| IBIS file useshx1xxac.ibs created by s2ibis3 verion 1.1
| North Carolina State University, ERL, 2006
| This Model is valid for Commercial Temperature Range 0C<=Tc<=95C
| Valid for DDR3-800/1066/1333/1600/1866 operation
| Part Number   VDD/VDDQ   Package   Architecture
| SCE15H1G160AF   1.5 +0.1/-0.1 96-Ball FBGA   64Meg x 16
| SCE15H1G800AF   1.5 +0.1/-0.1 78-Ball FBGA   128Meg x 8
| SCX15H512160AF   1.5 +0.1/-0.1 96-Ball FBGA   32Meg x 16
| SCX15H512800AF   1.5 +0.1/-0.1 78-Ball FBGA   64Meg x 8
[IBIS Ver]   3.2
[File name]  useshx1xxac.ibs
[File Rev]   1.2
[Date]   2016-10-26
[Source]   Simulation of a silicon level SPICE model
[Notes]   IBIS Characteristics for I/O Buffer
   IBIS Model Revision History:
Rev 1.1: 2014-07-22
   - IBIS model file initial creation
Rev 1.2: 2016-10-26
   - Updata company and other informations
   - Updata Rising/Falling Waveform for High speed
   - Updata power clamp of ODT_120/ODT_60/ODT_40/ODT_30/ODT_20
   - Updata package RLC value
[disclaimer] The IBIS models are for modeling purpose only and are
   subject to change without any notice. UniIC is not
   responsible for any problems the models may cause.
[Copyright]  Copyright 2009 UniIC Semiconductors Corp. All rights reserved
|   Component SCE15H1G160AF
[Component]   SCE15H1G160AF
[Manufacturer]  UniIC Semiconductors Corp.
| All balls excluding NC, POWER and GND (R[Ohm], L[H], C[F])
[Package]   | 96-Ball FBGA
|Variable   typ   min   max
R_pkg   4.62E-01   3.18E-01   5.65E-01
L_pkg   1.73E-09   1.10E-09   2.38E-09
C_pkg   5.30E-13   3.68E-13   7.38E-13
[Pin]   signal_name   model_name   R_pin   L_pin   C_pin
A1   VDDQ   POWER   NA   NA   NA
A2   DQU5   DQ   5.56E-01   1.93E-09   6.92E-13
A3   DQU7   DQ   4.86E-01   1.59E-09   6.10E-13
A7   DQU4   DQ   4.57E-01   1.38E-09   6.09E-13
A8   VDDQ   POWER   NA   NA   NA
A9   VSS   GND   NA   NA   NA
B1   VSSQ   GND   NA   NA   NA
B2   VDD   POWER   NA   NA   NA
B3   VSS   GND   NA   NA   NA
B7   DQSU#   DQ   5.07E-01   1.70E-09   5.10E-13
B8   DQU6   DQ   5.35E-01   1.74E-09   7.38E-13
B9   VSSQ   GND   NA   NA   NA
C1   VDDQ   POWER   NA   NA   NA
C2   DQU3   DQ   5.65E-01   1.76E-09   7.07E-13
C3   DQU1   DQ   4.98E-01   1.59E-09   6.47E-13
C7   DQSU   DQ   5.17E-01   1.87E-09   5.43E-13
C8   DQU2   DQ   4.97E-01   1.58E-09   5.57E-13
C9   VDDQ   POWER   NA   NA   NA
D1   VSSQ   GND   NA   NA   NA
D2   VDDQ   POWER   NA   NA   NA
D3   DMU   DM   4.84E-01   1.56E-09   6.30E-13
D7   DQU0   DQ   4.67E-01   1.57E-09   5.05E-13
D8   VSSQ   GND   NA   NA   NA
D9   VDD   POWER   NA   NA   NA
E1   VSS   GND   NA   NA   NA
E2   VSSQ   GND   NA   NA   NA
E3   DQL0   DQ   4.79E-01   1.40E-09   4.50E-13
E7   DML   DM   4.78E-01   1.54E-09   6.77E-13
E8   VSSQ   GND   NA   NA   NA
E9   VDDQ   POWER   NA   NA   NA
F1   VDDQ   POWER   NA   NA   NA
F2   DQL2   DQ   4.68E-01   1.62E-09   6.68E-13
F3   DQSL   DQ   4.57E-01   1.58E-09   4.57E-13
F7   DQL1   DQ   4.61E-01   1.63E-09   5.21E-13
F8   DQL3   DQ   5.04E-01   1.79E-09   6.87E-13
F9   VSSQ   GND   NA   NA   NA
G1   VSSQ   GND   NA   NA   NA
G2   DQL6   DQ   4.89E-01   1.50E-09   6.81E-13
G3   DQSL#   DQ   4.62E-01   1.55E-09   4.40E-13
G7   VDD   POWER   NA   NA   NA
G8   VSS   GND   NA   NA   NA
G9   VSSQ   GND   NA   NA   NA
H1   VREFDQ   POWER   NA   NA   NA
H2   VDDQ   POWER   NA   NA   NA
H3   DQL4   DQ   4.85E-01   1.58E-09   4.54E-13
H7   DQL7   DQ   4.57E-01   1.57E-09   4.72E-13
H8   DQL5   DQ   5.42E-01   1.77E-09   6.76E-13
H9   VDDQ   POWER   NA   NA   NA
J2   VSS   GND   NA   NA   NA
J3   RAS#   CLKCA_RCV   4.11E-01   1.55E-09   3.80E-13
J7   CK   CLKCA_RCV   4.24E-01   1.47E-09   3.68E-13
J8   VSS   GND   NA   NA   NA
K1   ODT   CLKCA_RCV   4.58E-01   1.94E-09   5.18E-13
K2   VDD   POWER   NA   NA   NA
K3   CAS#   CLKCA_RCV   3.18E-01   1.10E-09   4.11E-13
K7   CK#   CLKCA_RCV   4.31E-01   1.48E-09   3.87E-13
K8   VDD   POWER   NA   NA   NA
K9   CKE   CLKCA_RCV   4.57E-01   1.89E-09   4.77E-13
L2   CS#   CLKCA_RCV   4.36E-01   1.93E-09   5.07E-13
L3   WE#   CLKCA_RCV   4.32E-01   1.83E-09   4.90E-13
L7   A10   CLKCA_RCV   3.83E-01   1.62E-09   3.69E-13
L8   ZQ   NC   NA   NA   NA
M1   VSS   GND   NA   NA   NA
M2   BA0   CLKCA_RCV   4.00E-01   1.64E-09   4.95E-13
M3   BA2   CLKCA_RCV   4.44E-01   1.78E-09   4.47E-13
M8   VREFCA   POWER   NA   NA   NA
M9   VSS   GND   NA   NA   NA
N1   VDD   POWER   NA   NA   NA
N2   A3   CLKCA_RCV   4.56E-01   2.02E-09   4.33E-13
N3   A0   CLKCA_RCV   4.36E-01   1.84E-09   5.69E-13
N7   A12   CLKCA_RCV   3.99E-01   1.63E-09   5.01E-13
N8   BA1   CLKCA_RCV   4.64E-01   2.16E-09   4.55E-13
N9   VDD   POWER   NA   NA   NA
P1   VSS   GND   NA   NA   NA
P2   A5   CLKCA_RCV   4.19E-01   2.02E-09   5.57E-13
P3   A2   CLKCA_RCV   4.74E-01   1.94E-09   4.53E-13
P7   A1   CLKCA_RCV   4.35E-01   1.87E-09   4.43E-13
P8   A4   CLKCA_RCV   4.15E-01   1.88E-09   5.10E-13
P9   VSS   GND   NA   NA   NA
R1   VDD   POWER   NA   NA   NA
R2   A7   CLKCA_RCV   4.68E-01   1.94E-09   4.71E-13
R3   A9   CLKCA_RCV   4.27E-01   1.66E-09   5.18E-13
R7   A11   CLKCA_RCV   4.71E-01   1.94E-09   5.10E-13
R8   A6   CLKCA_RCV   4.71E-01   1.83E-09   4.71E-13
R9   VDD   POWER   NA   NA   NA
T1   VSS   GND   NA   NA   NA
T2   RESET#   CLKCA_RCV   4.79E-01   2.35E-09   7.31E-13
T3   A13   CLKCA_RCV   4.30E-01   1.76E-09   4.55E-13
T7   A14   CLKCA_RCV   4.33E-01   1.73E-09   5.40E-13
T8   A8   CLKCA_RCV   5.20E-01   2.38E-09   5.59E-13
T9   VSS   GND   NA   NA   NA
|*****************************  Diff Pin  *************************************
[Diff Pin]  inv_pin  vdiff   tdelay_typ  tdelay_min  tdelay_max
C7   B7   0.25000V   NA   NA   NA
F3   G3   0.25000V   NA   NA   NA
J7   K7   0.25000V   NA   NA   NA
|   Component SCE15H1G800AF
[Component]   SCE15H1G800AF
[Manufacturer]  UniIC Semiconductors Corp.
[Package]   | 78-Ball FBGA
|Variable   typ   min   max
R_pkg   3.88E-01   2.67E-01   5.49E-01
L_pkg   1.55E-09   1.21E-09   2.00E-09
C_pkg   5.15E-13   2.92E-13   7.34E-13
[Pin]   signal_name   model_name   R_pin   L_pin   C_pin
A1   VSS   GND   NA   NA   NA
A2   VDD   POWER   NA   NA   NA
A7   NU_TDQS#   NU_TDQS#   5.42E-01   1.89E-09   6.76E-13
A8   VSS   GND   NA   NA   NA
A9   VDD   POWER   NA   NA   NA
B1   VSS   GND   NA   NA   NA
B2   VSSQ   GND   NA   NA   NA
B3   DQ0   DQ   4.03E-01   1.53E-09   5.94E-13
B7   DM_TDQS   DM_TDQS   4.61E-01   1.83E-09   6.42E-13
B8   VSSQ   GND   NA   NA   NA
B9   VDDQ   POWER   NA   NA   NA
C1   VDDQ   POWER   NA   NA   NA
C2   DQ2   DQ   5.07E-01   1.89E-09   7.34E-13
C3   DQS   DQ   3.96E-01   1.55E-09   5.43E-13
C7   DQ1   DQ   4.34E-01   1.72E-09   5.27E-13
C8   DQ3   DQ   4.21E-01   1.77E-09   6.68E-13
C9   VSSQ   GND   NA   NA   NA
D1   VSSQ   GND   NA   NA   NA
D2   DQ6   DQ   5.49E-01   1.81E-09   6.19E-13
D3   DQS#   DQ   4.15E-01   1.63E-09   5.34E-13
D7   VDD   POWER   NA   NA   NA
D8   VSS   GND   NA   NA   NA
D9   VSSQ   GND   NA   NA   NA
E1   VREFDQ   POWER   NA   NA   NA
E2   VDDQ   POWER   NA   NA   NA
E3   DQ4   DQ   4.95E-01   1.56E-09   5.48E-13
E7   DQ7   DQ   4.13E-01   1.44E-09   4.60E-13
E8   DQ5   DQ   5.04E-01   1.56E-09   5.90E-13
E9   VDDQ   POWER   NA   NA   NA
F2   VSS   GND   NA   NA   NA
F3   RAS#   CLKCA_RCV   3.73E-01   1.42E-09   5.66E-13
F7   CK   CLKCA_RCV   3.22E-01   1.30E-09   4.89E-13
F8   VSS   GND   NA   NA   NA
G1   ODT   CLKCA_RCV   4.68E-01   2.00E-09   6.71E-13
G2   VDD   POWER   NA   NA   NA
G3   CAS#   CLKCA_RCV   3.75E-01   1.60E-09   4.41E-13
G7   CK#   CLKCA_RCV   3.24E-01   1.21E-09   4.51E-13
G8   VDD   POWER   NA   NA   NA
G9   CKE   CLKCA_RCV   4.14E-01   1.86E-09   7.10E-13
H2   CS#   CLKCA_RCV   3.75E-01   1.70E-09   5.45E-13
H3   WE#   CLKCA_RCV   3.53E-01   1.56E-09   3.77E-13
H7   A10   CLKCA_RCV   3.46E-01   1.38E-09   3.01E-13
H8   ZQ   NC   NA   NA   NA
J1   VSS   GND   NA   NA   NA
J2   BA0   CLKCA_RCV   3.35E-01   1.43E-09   5.84E-13
J3   BA2   CLKCA_RCV   3.55E-01   1.44E-09   5.18E-13
J8   VREFCA   POWER   NA   NA   NA
J9   VSS   GND   NA   NA   NA
K1   VDD   POWER   NA   NA   NA
K2   A3   CLKCA_RCV   3.89E-01   1.55E-09   4.28E-13
K3   A0   CLKCA_RCV   3.42E-01   1.52E-09   2.92E-13
K7   A12   CLKCA_RCV   3.25E-01   1.26E-09   4.48E-13
K8   BA1   CLKCA_RCV   3.14E-01   1.33E-09   4.58E-13
K9   VDD   POWER   NA   NA   NA
L1   VSS   GND   NA   NA   NA
L2   A5   CLKCA_RCV   3.29E-01   1.36E-09   4.52E-13
L3   A2   CLKCA_RCV   3.47E-01   1.59E-09   3.74E-13
L7   A1   CLKCA_RCV   3.45E-01   1.55E-09   4.31E-13
L8   A4   CLKCA_RCV   3.87E-01   1.46E-09   5.27E-13
L9   VSS   GND   NA   NA   NA
M1   VDD   POWER   NA   NA   NA
M2   A7   CLKCA_RCV   3.58E-01   1.50E-09   4.81E-13
M3   A9   CLKCA_RCV   3.32E-01   1.31E-09   3.74E-13
M7   A11   CLKCA_RCV   3.67E-01   1.54E-09   4.33E-13
M8   A6   CLKCA_RCV   3.71E-01   1.43E-09   5.17E-13
M9   VDD   POWER   NA   NA   NA
N1   VSS   GND   NA   NA   NA
N2   RESET#   CLKCA_RCV   2.67E-01   1.54E-09   6.32E-13
N3   A13   CLKCA_RCV   3.36E-01   1.31E-09   4.39E-13
N8   A8   CLKCA_RCV   3.43E-01   1.50E-09   5.05E-13
N9   VSS   GND   NA   NA   NA
|*****************************  Diff Pin  *************************************
[Diff Pin]  inv_pin  vdiff   tdelay_typ  tdelay_min  tdelay_max
F7   G7   0.25000V   NA   NA   NA
C3   D3   0.25000V   NA   NA   NA
|B7   A7   0.25000V   NA   NA   NA
|pin B7 and A7 are differential I/O only When TDQS/TDQS#
|is enabled via Mode Register A11=1 in MR1
|If TDQS is disabled, then B7 (DM) is a single
|ended INPUT with ODT and A7 is a NC
|   Component SCX15H512160AF
[Component]   SCX15H512160AF
[Manufacturer]  UniIC Semiconductors Corp.
| All balls excluding NC, POWER and GND (R[Ohm], L[H], C[F])
[Package]   | 96-Ball FBGA
|Variable   typ   min   max
R_pkg   4.62E-01   3.18E-01   5.65E-01
L_pkg   1.73E-09   1.10E-09   2.38E-09
C_pkg   5.30E-13   3.68E-13   7.38E-13
[Pin]   signal_name   model_name   R_pin   L_pin   C_pin
A1   VDDQ   POWER   NA   NA   NA
A2   DQU5   DQ   5.56E-01   1.93E-09   6.92E-13
A3   DQU7   DQ   4.86E-01   1.59E-09   6.10E-13
A7   DQU4   DQ   4.57E-01   1.38E-09   6.09E-13
A8   VDDQ   POWER   NA   NA   NA
A9   VSS   GND   NA   NA   NA
B1   VSSQ   GND   NA   NA   NA
B2   VDD   POWER   NA   NA   NA
B3   VSS   GND   NA   NA   NA
B7   DQSU#   DQ   5.07E-01   1.70E-09   5.10E-13
B8   DQU6   DQ   5.35E-01   1.74E-09   7.38E-13
B9   VSSQ   GND   NA   NA   NA
C1   VDDQ   POWER   NA   NA   NA
C2   DQU3   DQ   5.65E-01   1.76E-09   7.07E-13
C3   DQU1   DQ   4.98E-01   1.59E-09   6.47E-13
C7   DQSU   DQ   5.17E-01   1.87E-09   5.43E-13
C8   DQU2   DQ   4.97E-01   1.58E-09   5.57E-13
C9   VDDQ   POWER   NA   NA   NA
D1   VSSQ   GND   NA   NA   NA
D2   VDDQ   POWER   NA   NA   NA
D3   DMU   DM   4.84E-01   1.56E-09   6.30E-13
D7   DQU0   DQ   4.67E-01   1.57E-09   5.05E-13
D8   VSSQ   GND   NA   NA   NA
D9   VDD   POWER   NA   NA   NA
E1   VSS   GND   NA   NA   NA
E2   VSSQ   GND   NA   NA   NA
E3   DQL0   DQ   4.79E-01   1.40E-09   4.50E-13
E7   DML   DM   4.78E-01   1.54E-09   6.77E-13
E8   VSSQ   GND   NA   NA   NA
E9   VDDQ   POWER   NA   NA   NA
F1   VDDQ   POWER   NA   NA   NA
F2   DQL2   DQ   4.68E-01   1.62E-09   6.68E-13
F3   DQSL   DQ   4.57E-01   1.58E-09   4.57E-13
F7   DQL1   DQ   4.61E-01   1.63E-09   5.21E-13
F8   DQL3   DQ   5.04E-01   1.79E-09   6.87E-13
F9   VSSQ   GND   NA   NA   NA
G1   VSSQ   GND   NA   NA   NA
G2   DQL6   DQ   4.89E-01   1.50E-09   6.81E-13
G3   DQSL#   DQ   4.62E-01   1.55E-09   4.40E-13
G7   VDD   POWER   NA   NA   NA
G8   VSS   GND   NA   NA   NA
G9   VSSQ   GND   NA   NA   NA
H1   VREFDQ   POWER   NA   NA   NA
H2   VDDQ   POWER   NA   NA   NA
H3   DQL4   DQ   4.85E-01   1.58E-09   4.54E-13
H7   DQL7   DQ   4.57E-01   1.57E-09   4.72E-13
H8   DQL5   DQ   5.42E-01   1.77E-09   6.76E-13
H9   VDDQ   POWER   NA   NA   NA
J2   VSS   GND   NA   NA   NA
J3   RAS#   CLKCA_RCV   4.11E-01   1.55E-09   3.80E-13
J7   CK   CLKCA_RCV   4.24E-01   1.47E-09   3.68E-13
J8   VSS   GND   NA   NA   NA
K1   ODT   CLKCA_RCV   4.58E-01   1.94E-09   5.18E-13
K2   VDD   POWER   NA   NA   NA
K3   CAS#   CLKCA_RCV   3.18E-01   1.10E-09   4.11E-13
K7   CK#   CLKCA_RCV   4.31E-01   1.48E-09   3.87E-13
K8   VDD   POWER   NA   NA   NA
K9   CKE   CLKCA_RCV   4.57E-01   1.89E-09   4.77E-13
L2   CS#   CLKCA_RCV   4.36E-01   1.93E-09   5.07E-13
L3   WE#   CLKCA_RCV   4.32E-01   1.83E-09   4.90E-13
L7   A10   CLKCA_RCV   3.83E-01   1.62E-09   3.69E-13
L8   ZQ   NC   NA   NA   NA
M1   VSS   GND   NA   NA   NA
M2   BA0   CLKCA_RCV   4.00E-01   1.64E-09   4.95E-13
M3   BA2   CLKCA_RCV   4.44E-01   1.78E-09   4.47E-13
M8   VREFCA   POWER   NA   NA   NA
M9   VSS   GND   NA   NA   NA
N1   VDD   POWER   NA   NA   NA
N2   A3   CLKCA_RCV   4.56E-01   2.02E-09   4.33E-13
N3   A0   CLKCA_RCV   4.36E-01   1.84E-09   5.69E-13
N7   A12   CLKCA_RCV   3.99E-01   1.63E-09   5.01E-13
N8   BA1   CLKCA_RCV   4.64E-01   2.16E-09   4.55E-13
N9   VDD   POWER   NA   NA   NA
P1   VSS   GND   NA   NA   NA
P2   A5   CLKCA_RCV   4.19E-01   2.02E-09   5.57E-13
P3   A2   CLKCA_RCV   4.74E-01   1.94E-09   4.53E-13
P7   A1   CLKCA_RCV   4.35E-01   1.87E-09   4.43E-13
P8   A4   CLKCA_RCV   4.15E-01   1.88E-09   5.10E-13
P9   VSS   GND   NA   NA   NA
R1   VDD   POWER   NA   NA   NA
R2   A7   CLKCA_RCV   4.68E-01   1.94E-09   4.71E-13
R3   A9   CLKCA_RCV   4.27E-01   1.66E-09   5.18E-13
R7   A11   CLKCA_RCV   4.71E-01   1.94E-09   5.10E-13
R8   A6   CLKCA_RCV   4.71E-01   1.83E-09   4.71E-13
R9   VDD   POWER   NA   NA   NA
T1   VSS   GND   NA   NA   NA
T2   RESET#   CLKCA_RCV   4.79E-01   2.35E-09   7.31E-13
T3   A13   CLKCA_RCV   4.30E-01   1.76E-09   4.55E-13
T7   A14   CLKCA_RCV   4.33E-01   1.73E-09   5.40E-13
T8   A8   CLKCA_RCV   5.20E-01   2.38E-09   5.59E-13
T9   VSS   GND   NA   NA   NA
|*****************************  Diff Pin  *************************************
[Diff Pin]  inv_pin  vdiff   tdelay_typ  tdelay_min  tdelay_max
C7   B7   0.25000V   NA   NA   NA
F3   G3   0.25000V   NA   NA   NA
J7   K7   0.25000V   NA   NA   NA
|   Component SCX15H512800AF
[Component]   SCX15H512800AF
[Manufacturer]  UniIC Semiconductors Corp.
[Package]   | 78-Ball FBGA
|Variable   typ   min   max
R_pkg   3.88E-01   2.67E-01   5.49E-01
L_pkg   1.55E-09   1.21E-09   2.00E-09
C_pkg   5.15E-13   2.92E-13   7.34E-13
[Pin]   signal_name   model_name   R_pin   L_pin   C_pin
A1   VSS   GND   NA   NA   NA
A2   VDD   POWER   NA   NA   NA
A7   NU_TDQS#   NU_TDQS#   5.42E-01   1.89E-09   6.76E-13
A8   VSS   GND   NA   NA   NA
A9   VDD   POWER   NA   NA   NA
B1   VSS   GND   NA   NA   NA
B2   VSSQ   GND   NA   NA   NA
B3   DQ0   DQ   4.03E-01   1.53E-09   5.94E-13
B7   DM_TDQS   DM_TDQS   4.61E-01   1.83E-09   6.42E-13
B8   VSSQ   GND   NA   NA   NA
B9   VDDQ   POWER   NA   NA   NA
C1   VDDQ   POWER   NA   NA   NA
C2   DQ2   DQ   5.07E-01   1.89E-09   7.34E-13
C3   DQS   DQ   3.96E-01   1.55E-09   5.43E-13
C7   DQ1   DQ   4.34E-01   1.72E-09   5.27E-13
C8   DQ3   DQ   4.21E-01   1.77E-09   6.68E-13
C9   VSSQ   GND   NA   NA   NA
D1   VSSQ   GND   NA   NA   NA
D2   DQ6   DQ   5.49E-01   1.81E-09   6.19E-13
D3   DQS#   DQ   4.15E-01   1.63E-09   5.34E-13
D7   VDD   POWER   NA   NA   NA
D8   VSS   GND   NA   NA   NA
D9   VSSQ   GND   NA   NA   NA
E1   VREFDQ   POWER   NA   NA   NA
E2   VDDQ   POWER   NA   NA   NA
E3   DQ4   DQ   4.95E-01   1.56E-09   5.48E-13
E7   DQ7   DQ   4.13E-01   1.44E-09   4.60E-13
E8   DQ5   DQ   5.04E-01   1.56E-09   5.90E-13
E9   VDDQ   POWER   NA   NA   NA
F2   VSS   GND   NA   NA   NA
F3   RAS#   CLKCA_RCV   3.73E-01   1.42E-09   5.66E-13
F7   CK   CLKCA_RCV   3.22E-01   1.30E-09   4.89E-13
F8   VSS   GND   NA   NA   NA
G1   ODT   CLKCA_RCV   4.68E-01   2.00E-09   6.71E-13
G2   VDD   POWER   NA   NA   NA
G3   CAS#   CLKCA_RCV   3.75E-01   1.60E-09   4.41E-13
G7   CK#   CLKCA_RCV   3.24E-01   1.21E-09   4.51E-13
G8   VDD   POWER   NA   NA   NA
G9   CKE   CLKCA_RCV   4.14E-01   1.86E-09   7.10E-13
H2   CS#   CLKCA_RCV   3.75E-01   1.70E-09   5.45E-13
H3   WE#   CLKCA_RCV   3.53E-01   1.56E-09   3.77E-13
H7   A10   CLKCA_RCV   3.46E-01   1.38E-09   3.01E-13
H8   ZQ   NC   NA   NA   NA
J1   VSS   GND   NA   NA   NA
J2   BA0   CLKCA_RCV   3.35E-01   1.43E-09   5.84E-13
J3   BA2   CLKCA_RCV   3.55E-01   1.44E-09   5.18E-13
J8   VREFCA   POWER   NA   NA   NA
J9   VSS   GND   NA   NA   NA
K1   VDD   POWER   NA   NA   NA
K2   A3   CLKCA_RCV   3.89E-01   1.55E-09   4.28E-13
K3   A0   CLKCA_RCV   3.42E-01   1.52E-09   2.92E-13
K7   A12   CLKCA_RCV   3.25E-01   1.26E-09   4.48E-13
K8   BA1   CLKCA_RCV   3.14E-01   1.33E-09   4.58E-13
K9   VDD   POWER   NA   NA   NA
L1   VSS   GND   NA   NA   NA
L2   A5   CLKCA_RCV   3.29E-01   1.36E-09   4.52E-13
L3   A2   CLKCA_RCV   3.47E-01   1.59E-09   3.74E-13
L7   A1   CLKCA_RCV   3.45E-01   1.55E-09   4.31E-13
L8   A4   CLKCA_RCV   3.87E-01   1.46E-09   5.27E-13
L9   VSS   GND   NA   NA   NA
M1   VDD   POWER   NA   NA   NA
M2   A7   CLKCA_RCV   3.58E-01   1.50E-09   4.81E-13
M3   A9   CLKCA_RCV   3.32E-01   1.31E-09   3.74E-13
M7   A11   CLKCA_RCV   3.67E-01   1.54E-09   4.33E-13
M8   A6   CLKCA_RCV   3.71E-01   1.43E-09   5.17E-13
M9   VDD   POWER   NA   NA   NA
N1   VSS   GND   NA   NA   NA
N2   RESET#   CLKCA_RCV   2.67E-01   1.54E-09   6.32E-13
N8   A8   CLKCA_RCV   3.43E-01   1.50E-09   5.05E-13
N9   VSS   GND   NA   NA   NA
|*****************************  Diff Pin  *************************************
[Diff Pin]  inv_pin  vdiff   tdelay_typ  tdelay_min  tdelay_max
F7   G7   0.25000V   NA   NA   NA
C3   D3   0.25000V   NA   NA   NA
|B7   A7   0.25000V   NA   NA   NA
|pin B7 and A7 are differential I/O only When TDQS/TDQS#
|is enabled via Mode Register A11=1 in MR1
|If TDQS is disabled, then B7 (DM) is a single
|ended INPUT with ODT and A7 is a NC
|*****************************  Model Selector ********************************
[Model Selector]   DQ
DATA_34   RZQ/7 Output Driver (ODT Off)
DATA_40   RZQ/6 Output Driver (ODT Off)
DATA_80   RZQ/3 Output Driver (ODT Off)
DATA_60   RZQ/4 Output Driver (ODT Off)
DATA_RCV   Data/Data Strobe/Data Mask Receiver
ODT_60   ODT 60  Ohm (RZQ/4)
ODT_120   ODT 120 Ohm (RZQ/2)
ODT_40   ODT 40  Ohm (RZQ/6)
ODT_20   ODT 20  Ohm (RZQ/12)
ODT_30   ODT 30  Ohm (RZQ/8)
[Model Selector]   DM
DATA_RCV   Data/Data Strobe/Data Mask Receiver
ODT_60   ODT 60  Ohm (RZQ/4)
ODT_120   ODT 120 Ohm (RZQ/2)
ODT_40   ODT 40  Ohm (RZQ/6)
ODT_20   ODT 20  Ohm (RZQ/12)
ODT_30   ODT 30  Ohm (RZQ/8)
[Model Selector]   NU_TDQS#
DATA_NC   Non-Functioning Terminator Model
ODT_60   Data Strobe I/O with 60 Ohm ODT (RZQ/4)
ODT_120   Data Strobe I/O with 120 Ohm ODT (RZQ/2)
ODT_40   Data Strobe I/O with 40 Ohm ODT (RZQ/6)
ODT_20   Data Strobe I/O with 20 Ohm ODT (RZQ/12)
ODT_30   Data Strobe I/O with 30 Ohm ODT (RZQ/8)
|When TDQS# is enabled, NU_TDQS# is a output with terminal resistance;
|When TDQS# is disabled, NU_TDQS# is a NC;
[Model Selector]   DM_TDQS
DATA_RCV   Input Model with no ODT
ODT_60   Data Strobe I/O with 60 Ohm ODT (RZQ/4)
ODT_120   Data Strobe I/O with 120 Ohm ODT (RZQ/2)
ODT_40   Data Strobe I/O with 40 Ohm ODT (RZQ/6)
ODT_20   Data Strobe I/O with 20 Ohm ODT (RZQ/12)
ODT_30   Data Strobe I/O with 30 Ohm ODT (RZQ/8)
| Models and submodels in the file (12): DATA_34 (I/O), DATA_40 (I/O), DATA_80 (I/O), DATA_60 (I/O), DATA_RCV (Input), DATA_NC (Input), ODT_60 (Input), ODT_120 (Input), ODT_40 (Input), ODT_20 (Input), ODT_30 (Input), CLKCA_RCV (Input)
